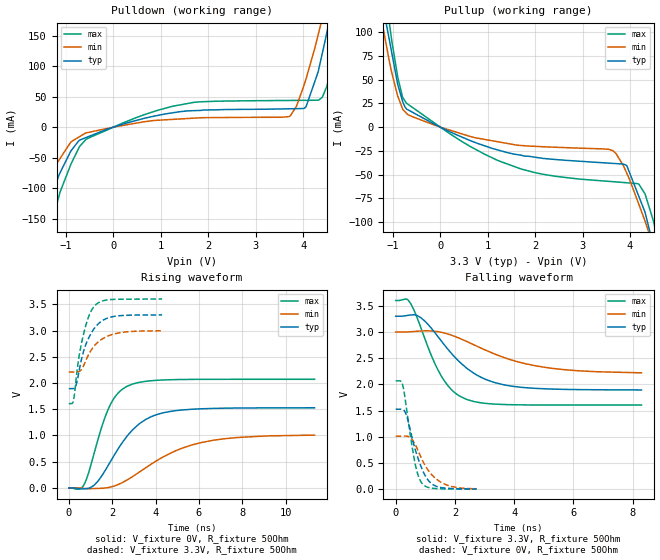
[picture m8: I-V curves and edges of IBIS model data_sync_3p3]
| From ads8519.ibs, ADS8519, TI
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|   data_sync_3p3 Model
[Model]   data_sync_3p3
Model_type   Output
Polarity   Non-Inverting
Vmeas = 1.65
Vref = 1.65
Cref = 5pF
Rref = 50
|   typ   min   max
|   (nom PVT)   (Fast PVT)   (slow PVT)
| C_comp by Frequency method (F=29Mhz)
|Average
|C_comp   1.178e-11   1.045e-11   1.327e-11
|ON state : BUFFER OUTPUT TURNED HIGH
|C_comp   1.178e-11   1.045e-11   1.327e-11
|OFF state: BUFFER OUTPUT TURNED LOW
|C_comp   1.082e-11   9.562e-12   1.188e-11
| C_comp by LC Tank method (L=1nH)
| Resonant frequency (Hz)  1.76e9   1.84e9   1.69e9
C_comp   8.158e-12   7.489e-12   8.846e-12
| Where nom  PVT is Nominal Process,  3.3V,  32C
|   Fast PVT is Strong Process,   3.6V,  -40C
|   Slow PVT is Weak Process,   3V,  92C
[Voltage Range]   3.3   3   3.6
|Ambient Temperature   25   85   -40
|Junction Temperature
[Temperature Range]   32   92   -40
[Pullup Reference]   3.3   3   3.6
[Pulldown Reference]   0   0   0
[Power Clamp Reference]   3.3   3   3.6
[GND Clamp Reference]   0   0   0
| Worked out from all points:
|   slope of the pulldown table from 0 to 0.495 V, typ, clamps not added: 43.8 ohm
|   slope of the pullup table from 0 to 0.495 V, typ, clamps not added: 43.7 ohm
|   falling waveform, V_fixture 3.3V, R_fixture 50Ohm: 20-80 % time 1.47ns typ, 2.23ns min, 953ps max; typ from 3.3 V to 1.9 V
|   rising waveform, V_fixture 0V, R_fixture 50Ohm: 20-80 % time 1.62ns typ, 2.7ns min, 1.01ns max; typ from 0 V to 1.53 V
|   rising waveform, V_fixture 3.3V, R_fixture 50Ohm: 20-80 % time 686ps typ, 817ps min, 542ps max; typ from 1.89 V to 3.3 V
|   falling waveform, V_fixture 0V, R_fixture 50Ohm: 20-80 % time 496ps typ, 647ps min, 348ps max; typ from 1.53 V to 0.007 V
[Pulldown]
|   Voltage   I(typ)   I(min)   I(max)
-3.3V     -584.4mA   -412.9mA   -810mA
-1.551V   -165.1mA   -110.6mA   -236mA
-1.336V   -118.9mA   -79.13mA   -166.9mA
-591mV    -17.51mA   -9.752mA   -21.13mA
1.246V    23.5mA     12.72mA    34.24mA
3.72V     30.13mA    17.97mA    43.83mA
4.059V    33.13mA    78.69mA    44mA
4.403V    120.9mA    179.3mA    48.9mA
4.507V    158.4mA    212.8mA    68.9mA
4.684V    226.4mA    270.2mA    136.6mA
5.098V    386.4mA    401.9mA    337.7mA
6.6V      902.2mA    846mA      986.5mA
[Pullup]
|   Voltage   I(typ)   I(min)   I(max)
-3.3V     870.5mA    742.1mA    1.056A
-1.213V   135.4mA    106.4mA    162.8mA
-1.068V   90.18mA    67.67mA    107.8mA
-896.4mV  44.76mA    32.59mA    52.57mA
-716.4mV  19.36mA    14.75mA    25.35mA
633.6mV   -14.25mA   -9.896mA   -20.46mA
2.012V    -31.85mA   -20.3mA    -48.17mA
3.636V    -38.24mA   -24.77mA   -57.51mA
3.93V     -40.42mA   -48.49mA   -58.68mA
4.187V    -73.19mA   -81.58mA   -60.21mA
4.468V    -120.5mA   -121.8mA   -94.96mA
6.6V      -628.2mA   -494mA     -776.4mA
[Ramp]
R_load = 50
|   typ   min   max
dV/dt_r   0.916646/1.61581e-09   0.607562/2.72074e-09   1.24242/1.005e-09
dV/dt_f   0.843858/1.47189e-09   0.473747/2.28867e-09   1.19615/9.5229e-10
[Falling Waveform]
V_fixture = 3.3V
V_fixture_min = 3V
V_fixture_max = 3.6V
R_fixture = 50Ohm
|   Time   V(typ)   V(min)   V(max)
0s        3.3V       3V         3.6V
495ps     3.323V     3.004V     3.552V
840ps     3.276V     3.018V     3.097V
1.515ns   2.846V     2.997V     2.184V
1.935ns   2.558V     2.928V     1.871V
2.37ns    2.322V     2.826V     1.72V
3.06ns    2.09V      2.647V     1.637V
3.96ns    1.964V     2.457V     1.613V
5.685ns   1.906V     2.281V     1.607V
8.295ns   1.895V     2.221V     1.606V
[Rising Waveform]
V_fixture = 0V
V_fixture_min = 0V
V_fixture_max = 0V
R_fixture = 50Ohm
|   Time   V(typ)   V(min)   V(max)
0s        2.612nV    3.03nV     2.328nV
495ps     -16.84mV   -1.573mV   -20.01mV
690ps     -16.2mV    -7.704mV   53.88mV
1.185ns   58.83mV    -10.93mV   686.1mV
1.8ns     417.4mV    6.148mV    1.482V
2.22ns    708.6mV    56.05mV    1.783V
2.775ns   1.03V      173.9mV    1.953V
4.065ns   1.399V     522.2mV    2.052V
6.12ns    1.509V     865.7mV    2.07V
11.34ns   1.528V     1.007V     2.071V
[Rising Waveform]
V_fixture = 3.3V
V_fixture_min = 3V
V_fixture_max = 3.6V
R_fixture = 50Ohm
|   Time   V(typ)   V(min)   V(max)
0s        1.894V     2.21V      1.606V
210ps     1.894V     2.21V      1.658V
360ps     1.996V     2.21V      2.164V
480ps     2.245V     2.222V     2.525V
630ps     2.527V     2.291V     2.843V
900ps     2.845V     2.531V     3.248V
1.185ns   3.046V     2.712V     3.467V
1.56ns    3.192V     2.844V     3.564V
2.025ns   3.264V     2.927V     3.593V
4.305ns   3.298V     2.995V     3.6V
[Falling Waveform]
V_fixture = 0V
V_fixture_min = 0V
V_fixture_max = 0V
R_fixture = 50Ohm
|   Time   V(typ)   V(min)   V(max)
0s        1.527V     1.014V     2.068V
165ps     1.527V     1.013V     2.064V
240ps     1.522V     1.014V     1.979V
375ps     1.391V     1.013V     1.502V
645ps     786.2mV    867.2mV    520.9mV
750ps     597.2mV    742.9mV    278.6mV
885ps     392.9mV    572.1mV    115.5mV
1.185ns   120mV      297.9mV    24.06mV
1.575ns   28.88mV    119.4mV    8.597mV
2.73ns    6.52mV     9.865mV    2.137mV
